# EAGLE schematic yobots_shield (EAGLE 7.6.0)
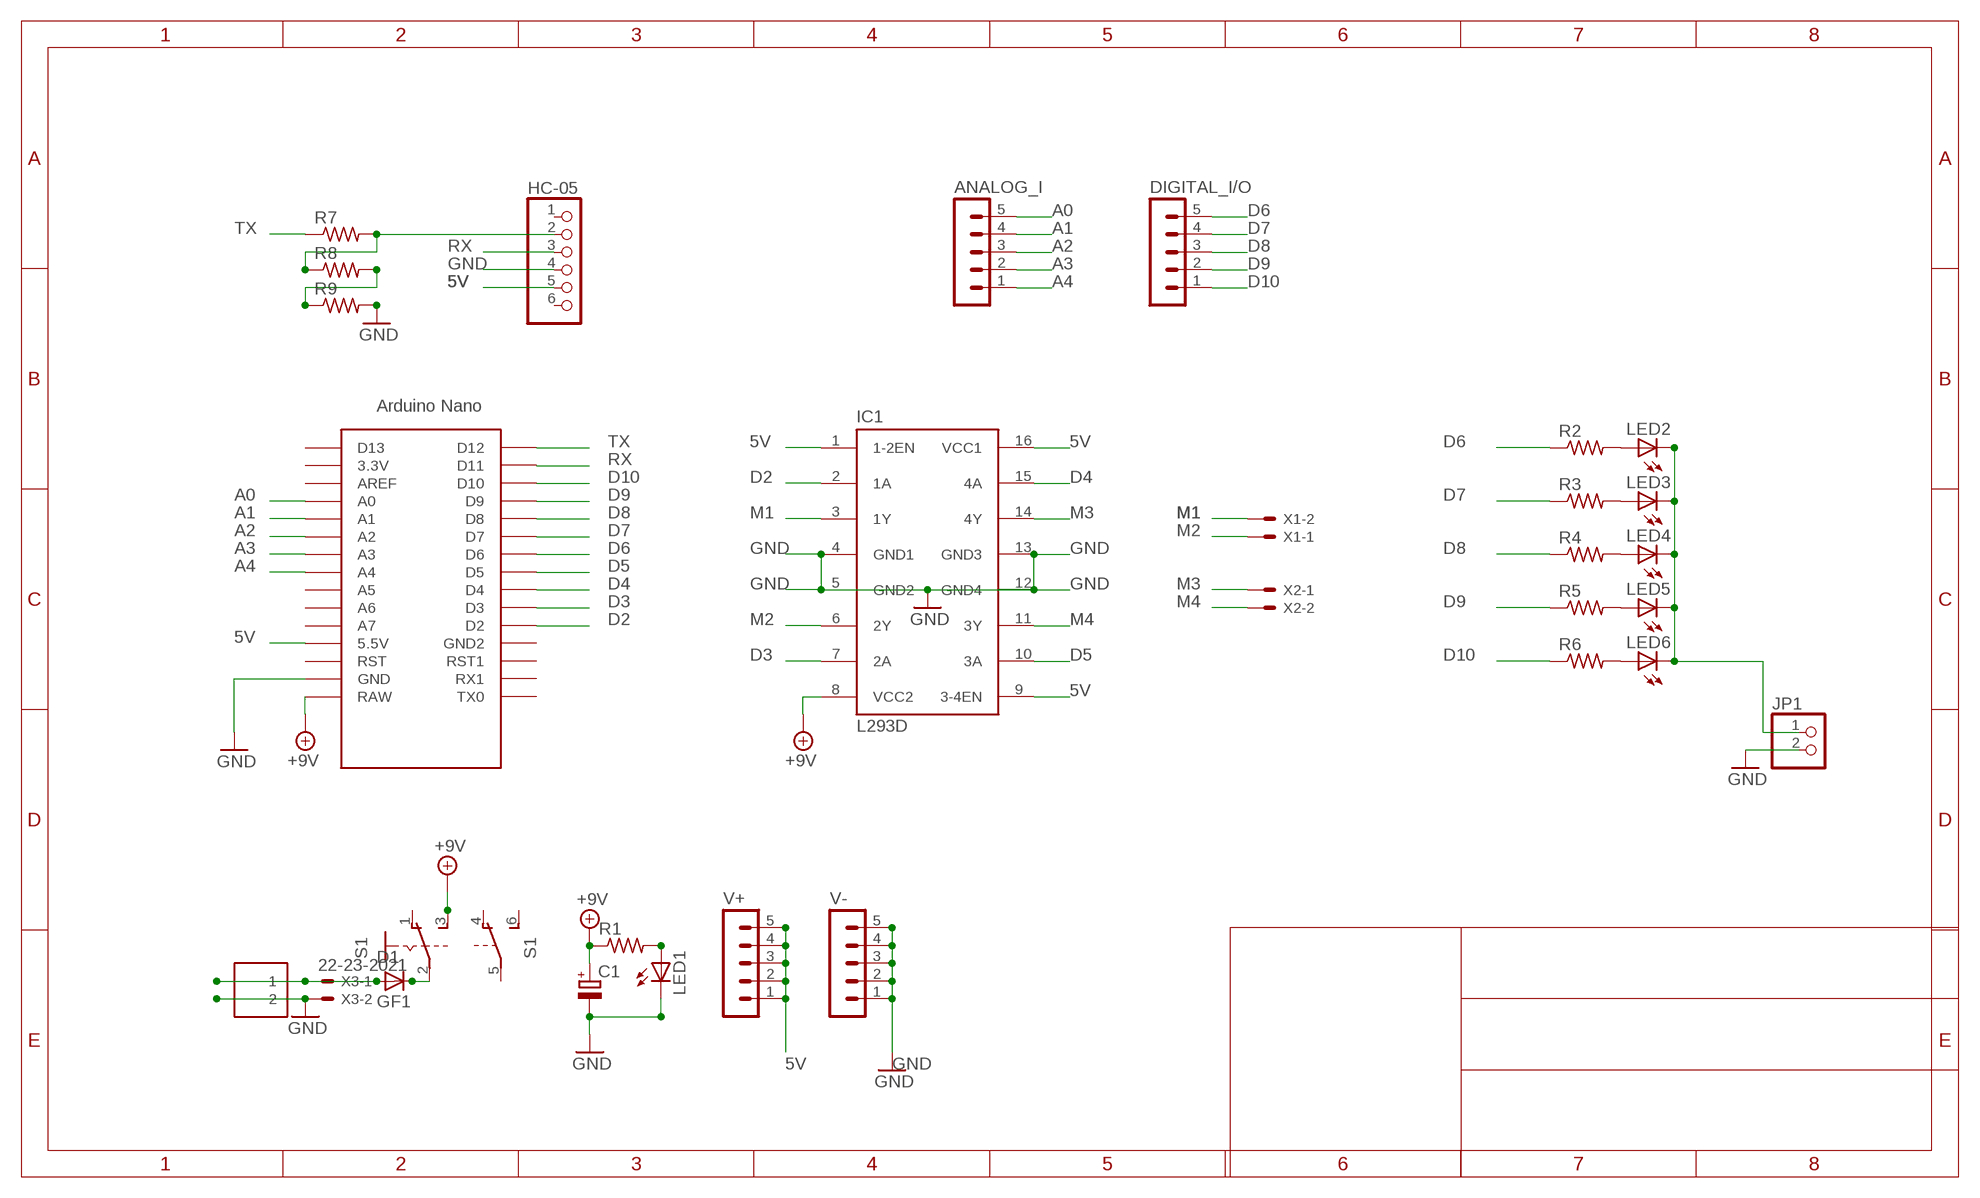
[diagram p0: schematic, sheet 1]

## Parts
ANALOG_I  MA05-1  [MA05-1]
C1  CPOL-EUD  [PANASONIC_D]
D1  GF1  [SMA-DO214AC]
DIGITAL_I/O  MA05-1  [MA05-1]
HC-05  PINHD-1X6  [1X06]
IC1  L293D  [DIL16]
J1  1X2-3.5MM  [1X2-3.5MM]
JP1  PINHD-1X2  [1X02]
LED1  LEDCHIPLED_1206  [CHIPLED_1206]
LED2  LEDCHIPLED_1206  [CHIPLED_1206]
LED3  LEDCHIPLED_1206  [CHIPLED_1206]
LED4  LEDCHIPLED_1206  [CHIPLED_1206]
LED5  LEDCHIPLED_1206  [CHIPLED_1206]
LED6  LEDCHIPLED_1206  [CHIPLED_1206]
R1  R-US_M1206  [M1206]
R2  R-US_M1206  [M1206]
R3  R-US_M1206  [M1206]
R4  R-US_M1206  [M1206]
R5  R-US_M1206  [M1206]
R6  R-US_M1206  [M1206]
R7  R-US_M1206  [M1206]
R8  R-US_M1206  [M1206]
R9  R-US_M1206  [M1206]
S1  A68-A31  [A68-A31]
U$1  NANO  [NANO]
V+  MA05-1  [MA05-1]
V-  MA05-1  [MA05-1]
X1  22-23-2021  [22-23-2021]
X2  22-23-2021  [22-23-2021]
X3  22-23-2021  [22-23-2021]

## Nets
5V: HC-05.5 IC1.1(1-2EN) IC1.9(3-4EN) IC1.16(VCC1) U$1.5V(5.5V) V+.1 V+.2 V+.3 V+.4 V+.5
+9V: C1.+ IC1.8(VCC2) R1.1 S1.3(A:S) U$1.RAW
A0: ANALOG_I.5 U$1.A0
A1: ANALOG_I.4 U$1.A1
A2: ANALOG_I.3 U$1.A2
A3: ANALOG_I.2 U$1.A3
A4: ANALOG_I.1 U$1.A4
D2: IC1.2(1A) U$1.D2
D3: IC1.7(2A) U$1.D3
D4: IC1.15(4A) U$1.D4
D5: IC1.10(3A) U$1.D5
D6: DIGITAL_I/O.5 R2.1 U$1.D6
D7: DIGITAL_I/O.4 R3.1 U$1.D7
D8: DIGITAL_I/O.3 R4.1 U$1.D8
D9: DIGITAL_I/O.2 R5.1 U$1.D9
D10: DIGITAL_I/O.1 R6.1 U$1.D10
GND: C1.- HC-05.4 IC1.4(GND1) IC1.5(GND2) IC1.12(GND4) IC1.13(GND3) J1.2 JP1.2 LED1.C R9.2 U$1.GND V-.1 V-.2 V-.3 V-.4 V-.5 X3.2
M1: IC1.3(1Y) X1.2
M2: IC1.6(2Y) X1.1
M3: IC1.14(4Y) X2.1
M4: IC1.11(3Y) X2.2
N$1: D1.A J1.1 X3.1
N$2: LED1.A R1.2
N$3: D1.K(C) S1.2(A:P)
N$4: LED2.A R2.2
N$5: LED3.A R3.2
N$6: LED4.A R4.2
N$7: HC-05.2 R7.2 R8.1
N$8: R8.2 R9.1
N$12: LED5.A R5.2
N$13: LED6.A R6.2
N$15: JP1.1 LED2.C LED3.C LED4.C LED5.C LED6.C
RX: HC-05.3 U$1.D11
TX: R7.1 U$1.D12
Unconnected: HC-05.1 HC-05.6 S1.1(A:O) S1.4(B:O) S1.5(B:P) S1.6(B:S) U$1.3.3V U$1.A5 U$1.A6 U$1.A7 U$1.AREF U$1.D13 U$1.GND1(GND2) U$1.ICSP1 U$1.ICSP2 U$1.ICSP3 U$1.ICSP4 U$1.ICSP5 U$1.ICSP6 U$1.RST U$1.RST1 U$1.RX1 U$1.TX0

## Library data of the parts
ANALOG_I DIGITAL_I/O V+ V- = con-lstb:MA05-1: PIN HEADER; OC_FARNELL: unknown; OC_NEWARK: unknown
C1 = rcl:CPOL-EU: POLARIZED CAPACITOR, European symbol
D1 = diode:GF1: DIODE
HC-05 = adafruit:PINHD-1X6: PIN HEADER
IC1 = st-microelectronics:L293D: PUSH-PULL 4 CHANNEL DRIVER; MPN: L293D; OC_FARNELL: 9589619; OC_NEWARK: 56P8249
J1 = adafruit:1X2: 3.5mm Terminal block
JP1 = pinhead:PINHD-1X2: PIN HEADER
LED1-LED6 = adafruit:LED: LED
R1-R9 = adafruit:R-US_: RESISTOR, American symbol
S1 = switch:A68-A31: SLIDING SWITCH Siemens, distributor Buerklin, 11G766
U$1 = Arduino-clone:NANO: Arduino Nano
X1-X3 = con-molex:22-23-2021: .100" (2.54mm) Center Header - 2 Pin; MF: MOLEX; MPN: 22-23-2021; OC_FARNELL: 1462926; OC_NEWARK: 25C3832

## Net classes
0 default: width 0.762 mm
